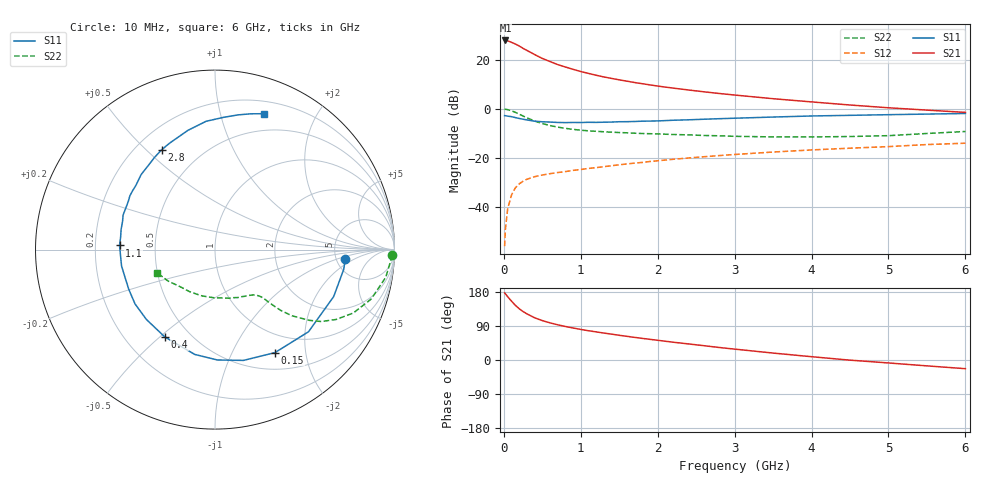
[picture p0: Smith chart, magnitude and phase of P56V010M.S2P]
! SIEMENS Small Signal Semiconductors
! BFP183
! Si NPN RF Bipolar Junction Transistor in SOT143
! VCE = 6 V  IC = 10 mA
! Common Emitter S-Parameters:  March  1996
# GHz  S  MA  R  50
!  f  S11  S21  S12  S22
! GHz  MAG  ANG  MAG  ANG  MAG  ANG  MAG  ANG
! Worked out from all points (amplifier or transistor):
!   36 points, 10 MHz to 6 GHz, reference 50 ohm
!   highest |S21| = 27.9 dB at 20 MHz (marker M1)
!   |S21| within 3 dB of that: start of sweep to 238.7 MHz
!   unconditionally stable (mu >= 1): 1.209 GHz to 5.649 GHz
!   at 250 MHz: K = 0.31, MSG = 27.1 dB, |S12| = -29.5 dB
!   at 1.4 GHz: K = 1.05, MAG = 16.4 dB, |S12| = -23.2 dB
!   at 6 GHz: K = 0.96, MSG = 6.3 dB, |S12| = -14.0 dB
!   lowest NFmin = 1.30 dB at 450 MHz
!   S11 on the Smith chart (normalised r, x): 10 MHz: 6.04, -1.34; 150 MHz: 0.72, -1.49; 400 MHz: 0.37, -0.52; 1.1 GHz: 0.31, +0.02; 2.8 GHz: 0.30, +0.56; 6 GHz: 0.32, +1.37
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0.01  0.7277 -4.1  24.57 177.2  0.0016 85.1  0.984 -1.8
0.02  0.7254 -8.8  24.71 174.9  0.0035 84.5  0.9807 -3.7
0.05  0.7111 -21.6  24.27 167.0  0.0093 81.8  0.9639 -9.2
0.1  0.6935 -41.3  22.59 155.2  0.0177 69.8  0.9125 -17.6
0.15  0.6641 -59.8  20.94 144.3  0.0247 63.1  0.8481 -24.6
0.2  0.6374 -75.6  19.04 135.3  0.0297 57.4  0.7787 -30.0
0.25  0.615 -88.8  17.06 127.8  0.0336 52.4  0.7149 -34.1
0.3  0.5949 -100.9  15.5 121.8  0.0369 49.6  0.6562 -36.9
0.4  0.5612 -119.9  12.75 111.4  0.0416 45.0  0.5653 -40.7
0.5  0.5455 -134.5  10.63 104.0  0.045 42.2  0.5017 -42.7
0.6  0.5386 -145.8  9.197 98.0  0.0479 41.5  0.4575 -43.6
0.7  0.529 -155.2  7.971 92.9  0.0505 41.8  0.4248 -44.3
0.9  0.5286 -170.1  6.386 84.5  0.0559 41.5  0.3822 -45.1
1.1  0.5324 177.5  5.27 77.2  0.0613 42.0  0.3569 -46.4
1.5  0.5471 159.4  3.897 65.2  0.0727 42.9  0.3296 -50.0
1.8  0.561 147.7  3.25 57.0  0.0811 43.0  0.3146 -54.3
2.2  0.5865 134.6  2.648 47.0  0.0939 41.6  0.3005 -60.9
2.8  0.6304 118.2  2.056 33.0  0.1119 38.5  0.2828 -73.4
3.5  0.6813 102.8  1.61 18.3  0.1321 34.6  0.2685 -90.9
4.5  0.7381 86.4  1.198 -0.4  0.1581 27.3  0.2734 -120.5
5.5  0.7826 75.2  0.943 -15.5  0.1876 20.8  0.3153 -146.4
6  0.8046 70.2  0.847 -22.9  0.1999 16.5  0.3461 -157.9
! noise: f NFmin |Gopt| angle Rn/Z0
0.45  1.3  0.15  45  0.18
0.9  1.4  0.2  125  0.19
1.8  2.1  0.34  -170  0.14
